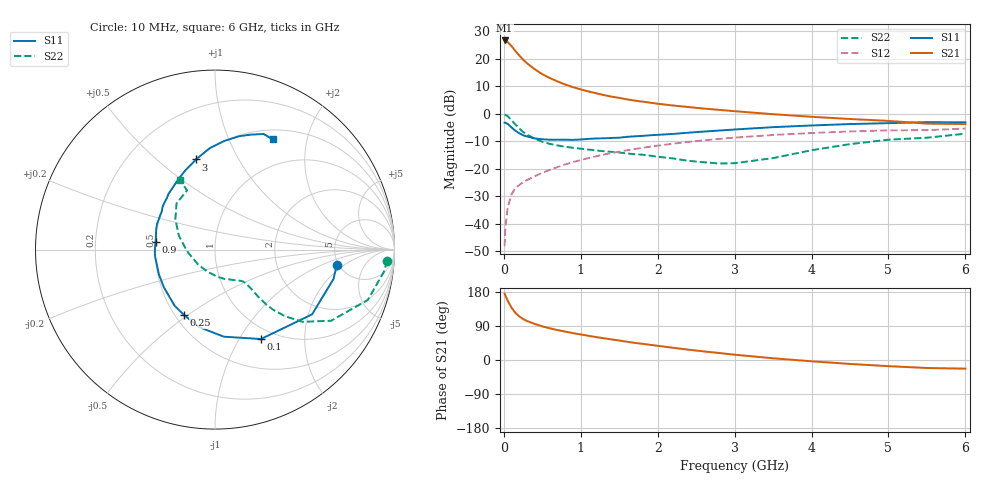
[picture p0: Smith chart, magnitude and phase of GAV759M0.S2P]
! Infineon Technologies  Discrete & RF Semiconductors
! BF775
! Si NPN RF Bipolar Junction Transistor in SOT23
! VCE = 0.75 V  IC = 9 mA
! Common Emitter S-Parameters:  May  1996
# GHz  S  MA  R  50
!  f  S11  S21  S12  S22
! GHz  MAG  ANG  MAG  ANG  MAG  ANG  MAG  ANG
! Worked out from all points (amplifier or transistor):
!   36 points, 10 MHz to 6 GHz, reference 50 ohm
!   highest |S21| = 26.6 dB at 10 MHz (marker M1)
!   |S21| within 3 dB of that: start of sweep to 126.5 MHz
!   unconditionally stable (mu >= 1): 465.7 MHz to end of sweep
!   at 250 MHz: K = 0.73, MSG = 22.3 dB, |S12| = -25.0 dB
!   at 1.4 GHz: K = 1.20, MAG = 7.6 dB, |S12| = -14.3 dB
!   at 6 GHz: K = 1.06, MAG = -0.6 dB, |S12| = -5.4 dB
!   S11 on the Smith chart (normalised r, x): 10 MHz: 4.80, -1.57; 100 MHz: 0.86, -1.24; 250 MHz: 0.56, -0.48; 900 MHz: 0.50, +0.05; 3 GHz: 0.50, +0.68; 6 GHz: 0.62, +1.47
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0.01  0.6839 -7.3  21.3 175.1  0.0039 85.9  0.9619 -3.7
0.02  0.6802 -13.9  21.06 170.1  0.0087 80.4  0.9479 -7.7
0.05  0.6503 -33.7  19.93 156.5  0.0195 74.6  0.896 -18.3
0.1  0.5601 -62.8  16.82 137.9  0.0343 64.1  0.7585 -31.5
0.15  0.4878 -84.2  13.69 124.4  0.044 57.5  0.6326 -39.5
0.2  0.4407 -101.5  11.38 115.2  0.0503 55.6  0.5378 -43.6
0.25  0.4033 -115.4  9.56 108.1  0.0564 54.8  0.4647 -46.0
0.3  0.3852 -125.8  8.234 103.0  0.0618 55.4  0.4142 -47.0
0.4  0.3537 -143.8  6.413 95.3  0.0729 56.1  0.3506 -47.5
0.5  0.3418 -156.1  5.196 88.8  0.0838 57.4  0.3079 -47.3
0.6  0.3348 -165.7  4.407 83.5  0.0954 58.4  0.2809 -47.3
0.7  0.3364 -174.6  3.825 78.9  0.1072 59.1  0.2633 -47.4
0.9  0.3335 172.8  3.02 70.9  0.1318 58.8  0.2388 -48.5
1.1  0.3468 161.0  2.527 63.8  0.1554 58.0  0.2221 -51.5
1.3  0.3555 152.1  2.17 57.3  0.18 56.4  0.2072 -54.9
1.6  0.3781 140.4  1.811 48.2  0.2153 53.5  0.1888 -62.4
2.2  0.427 121.4  1.401 32.3  0.2838 46.1  0.1532 -84.3
3  0.5135 101.9  1.105 14.0  0.3661 34.9  0.1254 -138.6
3.5  0.5665 92.9  0.974 4.5  0.4079 27.7  0.1554 -176.3
4.5  0.6452 78.1  0.797 -10.4  0.4735 13.9  0.2788 142.4
5.5  0.6988 67.2  0.657 -21.1  0.4997 0.6  0.3645 115.3
6  0.6935 62.4  0.645 -22.8  0.535 -3.2  0.4315 116.7
